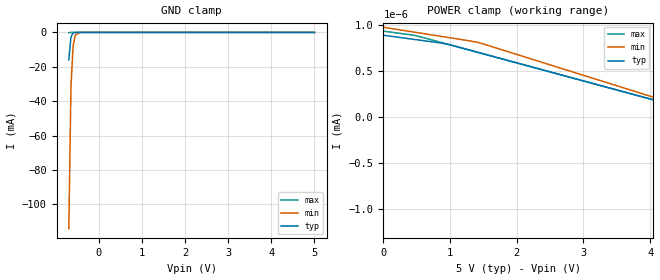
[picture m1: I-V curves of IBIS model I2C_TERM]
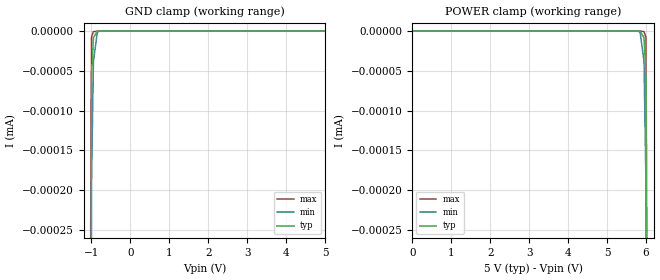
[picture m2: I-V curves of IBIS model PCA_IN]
|   NXP Semiconductors Inc.
|   Specialty Logic Products Group
|   IBIS model of PCA9546A
|   4-Channel I2C switch with reset
[IBIS Ver]   3.2
[Comment Char]   |_char
| VDD TYP:5V, MIN:4.5V, MAX: 5.5V
[File name]   pca9546a_5v.ibs
[File Rev]   1.0
[Date]   Dec 14, 2007 10:28:50 AM
[Source]
Generated by Seshadri Venkataramanan with IbisToolKit at Tempe, AZ
[Notes]
[Disclaimer]
(C) Copyright 2007 NXP Semiconductors
All rights reserved
NXP Semiconductors (NXP) does not warrant that this model and any other
accompanying information (Model) accurately or fully represents the
operating characteristics and specifications of the semiconductor
products to which the Model relates.  Moreover, the Model is furnished
on an "as is" and with "all faults" basis, and without support or
warranty of any kind.  NXP disclaims all warranties, whether expressed
or implied or statutory, including without limitation all implied
warranties of non-infringement, merchantability and fitness for any
purpose, and those arising from a course of dealing or usage of trade.
NXP does not convey any license under its or any third party's patents,
copyrights or other intellectual property or proprietary rights.
You and your company assume any and all risks and liability arising out
of the application or use of the Model.
In no event shall NXP be liable for any direct, indirect, special,
consequential or incidental damages, however caused, whether in
warranty, contract or tort (including negligence), strict liability or
other legal theory, including, without limitation, for lost profits,
business interruption, or corruption or loss of data or information,
arising out of or in connection with the use of or the inability to use
the Model, even if NXP has been advised of the possibility of such
damages.
NXP provides the Model as a courtesy to our customers. You and your
company shall not distribute, convey, sell, or give the Model to anyone
else without receiving prior written permission from NXP.
NXP reserves the right to make changes without notice to the Model to
improve reliability, function, or design.
Please be aware that your receipt and subsequent use of the Model shall
serve as acceptance of these terms and conditions.  If you do not
accept these terms, return or destroy the Model immediately.
[Copyright]
2007
[Component]   PCA9546AD
Si_location Pin
Timing_location Pin
[Manufacturer]   NXP Semiconductors
[Package]
|   variable   typ   min   max
R_pkg   1.75E-01   1.28E-01   2.11E-01
L_pkg   5.03E-09   3.94E-09   6.26E-09
C_pkg   0.794E-12   0.715E-12   0.869E-12
|  SO16
[Pin] signal_name   model_name   R_pin   L_pin   C_pin
1   A0   PCA_IN   1.99E-01  6.26E-09  0.822E-12
2   A1   PCA_IN   2.11E-01  5.46E-09  0.869E-12
3   RESETB   PCA_IN   1.56E-01  4.44E-09  0.760E-12
4   SD0   I2C_TERM   1.28E-01  3.94E-09  0.717E-12
5   SC0   I2C_TERM   1.28E-01  3.94E-09  0.715E-12
6   SD1   I2C_TERM   1.56E-01  4.44E-09  0.760E-12
7   SC1   I2C_TERM   2.11E-01  5.46E-09  0.869E-12
8   Vss   GND   1.99E-01  6.26E-09  0.843E-12
9   SD2   I2C_TERM   1.99E-01  6.26E-09  0.843E-12
10   SC2   I2C_TERM   2.11E-01  5.46E-09  0.869E-12
11   SD3   I2C_TERM   1.56E-01  4.44E-09  0.760E-12
12   SC3   I2C_TERM   1.28E-01  3.94E-09  0.717E-12
13   A2   PCA_IN   1.28E-01  3.94E-09  0.715E-12
14   SCL   I2C_TERM   1.56E-01  4.44E-09  0.760E-12
15   SDA   I2C_TERM   2.11E-01  5.46E-09  0.869E-12
16   Vdd   POWER   1.99E-01  6.26E-09  0.843E-12
[Series Pin Mapping] pin_2 model_name   function_table_group
14   5   PCA_SW   1
14   7   PCA_SW   2
14   10   PCA_SW   3
14   12   PCA_SW   4
15   6   PCA_SW   2
15   4   PCA_SW   1
15   11   PCA_SW   4
15   9   PCA_SW   3
[Series Switch Groups]
Off 1 2 3 4 /
On 1 /
On 2 /
On 3 /
On 4 /
[Component]   PCA9546APW
Si_location Pin
Timing_location Pin
[Manufacturer]   NXP Semiconductors
[Package]
|   variable   typ   min   max
R_pkg   3.44E-02   2.80E-02   4.33E-02
L_pkg   1.83E-09   1.36E-09   2.32E-09
C_pkg   0.380E-12   0.302E-12   0.442E-12
|  TSSOP16
[Pin] signal_name   model_name   R_pin   L_pin   C_pin
1   A0   PCA_IN   3.52E-02  2.40E-09  0.436E-12
2   A1   PCA_IN   3.70E-02  1.93E-09  0.438E-12
3   RESETB   PCA_IN   4.56E-02  1.76E-09  0.345E-12
4   SD0   I2C_TERM   4.00E-02  1.65E-09  0.335E-12
5   SC0   I2C_TERM   4.00E-02  1.65E-09  0.335E-12
6   SD1   I2C_TERM   4.56E-02  1.76E-09  0.345E-12
7   SC1   I2C_TERM   3.70E-02  1.93E-09  0.438E-12
8   Vss   GND   3.52E-02  2.40E-09  0.452E-12
9   SD2   I2C_TERM   3.52E-02  2.40E-09  0.452E-12
10   SC2   I2C_TERM   3.70E-02  1.93E-09  0.438E-12
11   SD3   I2C_TERM   4.56E-02  1.76E-09  0.345E-12
12   SC3   I2C_TERM   4.00E-02  1.65E-09  0.771E-12
13   A2   PCA_IN   4.00E-02  1.65E-09  0.771E-12
14   SCL   I2C_TERM   4.56E-02  1.76E-09  0.345E-12
15   SDA   I2C_TERM   3.70E-02  1.93E-09  0.438E-12
16   Vdd   POWER   3.52E-02  2.40E-09  0.452E-12
[Series Pin Mapping] pin_2 model_name   function_table_group
14   5   PCA_SW   1
14   7   PCA_SW   2
14   10   PCA_SW   3
14   12   PCA_SW   4
15   4   PCA_SW   1
15   6   PCA_SW   2
15   9   PCA_SW   3
15   11   PCA_SW   4
[Series Switch Groups]
Off 1 2 3 4 /
On 1 /
On 2 /
On 3 /
On 4 /
[Component]   PCA9546ABS
Si_location Pin
Timing_location Pin
[Manufacturer]   NXP Semiconductors
[Package]
|   [Package]   HVQFN16 (uses tssop24 data here only)
|   variable   typ   min   max
R_pkg   3.44E-02   2.80E-02   4.33E-02
L_pkg   1.83E-09   1.36E-09   2.32E-09
C_pkg   0.380E-12   0.302E-12   0.442E-12
|  HVQFN16
[Package Model]   hvqfn16
[Pin] signal_name   model_name
1   RESETB   PCA_IN
2   SD0   I2C_TERM
3   SC0   I2C_TERM
4   SD1   I2C_TERM
5   SC1   I2C_TERM
6   Vss   GND
7   SD2   I2C_TERM
8   SC2   I2C_TERM
9   SD3   I2C_TERM
10   SC3   I2C_TERM
11   A2   I2C_TERM
12   SCL   I2C_TERM
13   SDA   I2C_TERM
14   Vdd   POWER
15   A0   PCA_IN
16   A1   PCA_IN
[Series Pin Mapping] pin_2 model_name   function_table_group
12   3   PCA_SW   1
12   5   PCA_SW   2
12   8   PCA_SW   3
12   10   PCA_SW   4
13   2   PCA_SW   1
13   4   PCA_SW   2
13   7   PCA_SW   3
13   9   PCA_SW   4
[Series Switch Groups]
|   Function Group States
| default
Off 1 2 3 4 /
On 1 /
On 2 /
On 3 /
On 4 /
| [End   I2C_TERM
[Define Package Model]   hvqfn16
[Manufacturer]   Unknown
[OEM]   Unknown
[Description]   For pca9544a and pca9545a
[Number of Pins]   16
[Pin Numbers]
|   1 = D2
1
|   2 = D3
2
|   3 = D4
3
|   4 = D5
4
|   5 = D6
5
|   6 = D7
6
|   7 = NC
7
|   8 = Vss
8
|   9 = WRn
9
|   10 = RDn
10
|   11 = CEn
11
|   12 = A0
12
|   13 = A1
13
|   14 = INTn
14
|   15 = RESETn
15
|   16 = SCL
16
|   17 = SDA
|   18 = Vdd
|   19 = D0
|   20 = D1
[Model Data]
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[End Model Data]
[End Package Model]
[Model]   PCA_SW
Model_type Series_switch
C_comp   2.51p   2.51p   2.51p
[Temperature Range] 27   85   -40
[Voltage Range]   5   4.5   5.5
[Pullup Reference]  5   4.5   5.5
[Pulldown Reference]0   0   0
[On]
[R Series]   9   4   24
[L Series]   1n   1n   1n
[C Series]   1p   1p   1p
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[Off]
|   variable   R(typ)   R(min)   R(max)
[R Series]   1e06   1e06   1e06
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| Models and submodels in the file (3): I2C_TERM (Terminator), PCA_IN (Input), PCA_SW (Series_switch)
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[Model]   I2C_TERM
Model_type Terminator
C_comp   9.5p   9.5p   9.5p
[Temperature Range] 27   85   -40
[Voltage Range]   5   4.5   5.5
[Pullup Reference]  5   4.5   5.5
[Pulldown Reference]5   4.5   5.5
[POWER Clamp Reference]5   4.5   5.5
[GND Clamp Reference]0   0   0
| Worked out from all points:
|   GND clamp passes 1 mA (typ) near -0.61 V on its own axis
[GND Clamp]
|   -6.000000E-1   -1.554225E-1   -1.242642E-1   -2.666059E-1
|   -5.000000E-1   -1.602113E-1   -1.179351E-1   -2.662641E-1
|   -4.000000E-1   -1.574088E-1   -1.099432E-1   -2.800035E-1
-700mV    -15.98mA   -114.2mA   -166.1uA
-650mV    -2.657mA   -31.47mA   -13.81uA
-600mV    -395.8uA   -7.677mA   -1.147uA
-550mV    -57.53uA   -1.648mA   -95.33nA
-450mV    -1.205uA   -66.13uA   -744.9pA
-400mV    -174.5nA   -13.1uA    -133.3pA
5V        893.1pA    979.7pA    937.7pA
[POWER Clamp]
0V        893.1pA    979.7pA    937.7pA
5V        0A         0A         0A
5.05V     -10.05pA   -134.7pA   -9.85pA
5.1V      -21.27pA   -775.2pA   -19.7pA
5.2V      -115.8pA   -20.09nA   -39.4pA
5.25V     -577.4pA   -101.5nA   -49.28pA
5.3V      -3.71nA    -512.9nA   -59.48pA
5.35V     -25.3nA    -2.592uA   -73.47pA
5.4V      -174.5nA   -13.1uA    -133.3pA
5.45V     -1.205uA   -66.13uA   -744.9pA
5.55V     -57.53uA   -1.648mA   -95.33nA
5.7V      -15.98mA   -114.2mA   -166.1uA
[Model]   PCA_IN
Model_type Input
Vinh=2.1
Vinl=0.9
C_comp   1.73p   1.73p   1.73p
[Temperature Range] 27   85   -40
[Voltage Range]   5   4.5   5.5
[POWER Clamp Reference]5   4.5   5.5
[GND Clamp Reference]0   0   0
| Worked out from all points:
|   GND clamp passes 1 mA (typ) near -1.21 V on its own axis
[GND Clamp]
-2V       -10.17A    -9.093A    -11.52A
-1.1V     -2.718uA   -4.916uA   -1.14uA
-1V       -56.9nA    -192.5nA   -7.858nA
-950mV    -8.234nA   -38.09nA   -653.2pA
-850mV    -173.2pA   -1.492nA   -5.345pA
-800mV    -25.74pA   -295.9pA   -1.173pA
5V        5pA        5pA        5pA
[POWER Clamp]
0V        5pA        5pA        5pA
5.8V      -25.74pA   -295.9pA   -1.173pA
5.85V     -173.2pA   -1.492nA   -5.345pA
5.95V     -8.234nA   -38.09nA   -653.2pA
6V        -56.9nA    -192.5nA   -7.858nA
6.1V      -2.718uA   -4.916uA   -1.14uA
7V        -10.17A    -9.093A    -11.52A
